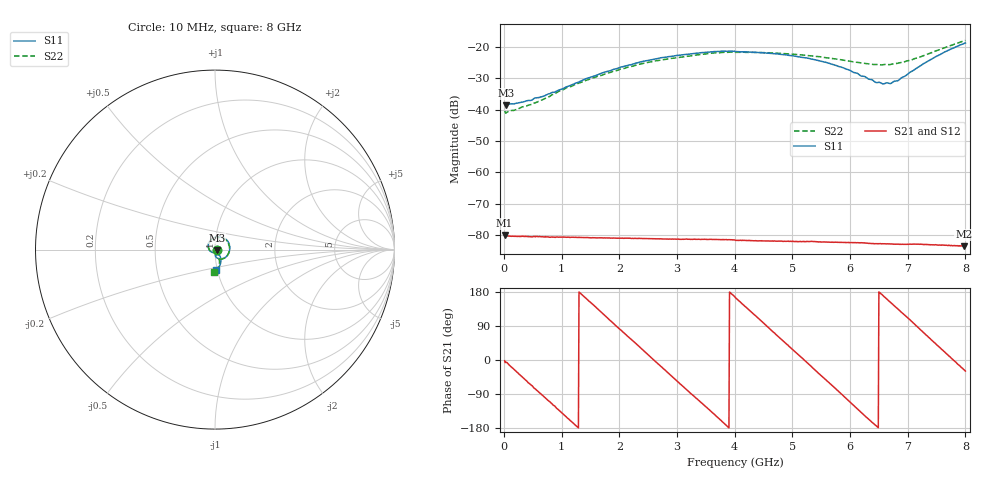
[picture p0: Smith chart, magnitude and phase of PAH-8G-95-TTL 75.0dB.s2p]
! MTS Systemtechnik GmbH
! S-Parameters
! Model: PAH-8G/95-TTL
! Attenuation Step: 75.0dB
! Rohde & Schwarz ZVB8 2Ports - Version 4.11 - 1145.1010k08 SN: 100119
! S2P File Measurements:
! S11 S21 S12 S22
# HZ  S  DB  R  50.00
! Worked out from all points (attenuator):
!   800 points, 10 MHz to 8 GHz, reference 50 ohm
!   highest |S21| = -80.08 dB at 10 MHz (marker M1); lowest = -83.6 dB at 7.97 GHz (marker M2)
!   lowest |S11| = -38.7 dB at 30 MHz (marker M3), VSWR 1.02, Z = 51.2 - j0.178 ohm
!   |S11| at or under -10 dB: start of sweep to end of sweep
!   |S22| runs from -41.2 to -17.9 dB; largest |S21 - S12| = 2.4e-06
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1e7  -38.07 -10.3  -80.08 -2.0  -79.89 -1.7  -40.52 -12.8
3e7  -38.69 -8.6  -80.41 -5.8  -80.36 -5.7  -41.16 -10.3
2e8  -38.05 -28.4  -80.45 -28.6  -80.48 -28.5  -40.07 -32.1
3.1e8  -37.65 -43.5  -80.46 -43.9  -80.47 -44.0  -39.17 -48.5
6.6e8  -35.89 -90.4  -80.59 -92.3  -80.52 -92.7  -36.92 -96.4
1.08e9  -32.76 -139.4  -80.76 -150.1  -80.76 -149.9  -33.05 -141.1
1.35e9  -30.76 -166.1  -80.81 172.4  -80.85 172.5  -31.19 -164.9
2.03e9  -26.42 140.7  -81.06 78.4  -81.06 78.4  -27.03 143.9
2.68e9  -23.64 98.0  -81.26 -11.3  -81.24 -11.1  -24.33 103.0
3.43e9  -21.84 53.9  -81.42 -114.0  -81.46 -114.0  -22.38 59.0
4.01e9  -21.50 19.4  -81.72 164.9  -81.78 164.8  -21.74 26.2
4.71e9  -22.20 -20.3  -82.02 68.0  -82.00 68.2  -22.01 -10.9
5.34e9  -23.91 -54.1  -82.06 -19.0  -82.15 -18.8  -22.88 -40.7
5.87e9  -26.60 -77.8  -82.38 -92.6  -82.42 -92.5  -24.21 -60.2
6.45e9  -31.37 -81.8  -82.81 -173.2  -82.84 -173.5  -25.61 -69.7
6.57e9  -31.80 -75.6  -82.84 170.3  -82.81 170.4  -25.69 -69.8
6.67e9  -31.61 -68.0  -82.89 155.9  -82.85 156.4  -25.68 -68.5
6.83e9  -30.77 -59.4  -82.96 134.4  -83.04 134.4  -25.20 -68.2
7.06e9  -27.94 -52.5  -82.98 102.9  -82.92 103.0  -24.20 -67.8
7.49e9  -23.05 -61.7  -83.17 42.4  -83.21 41.7  -21.28 -73.7
7.97e9  -18.95 -84.5  -83.60 -25.1  -83.66 -24.7  -18.07 -90.2
8e9  -18.75 -86.0  -83.58 -29.1  -83.69 -28.8  -17.95 -91.6
